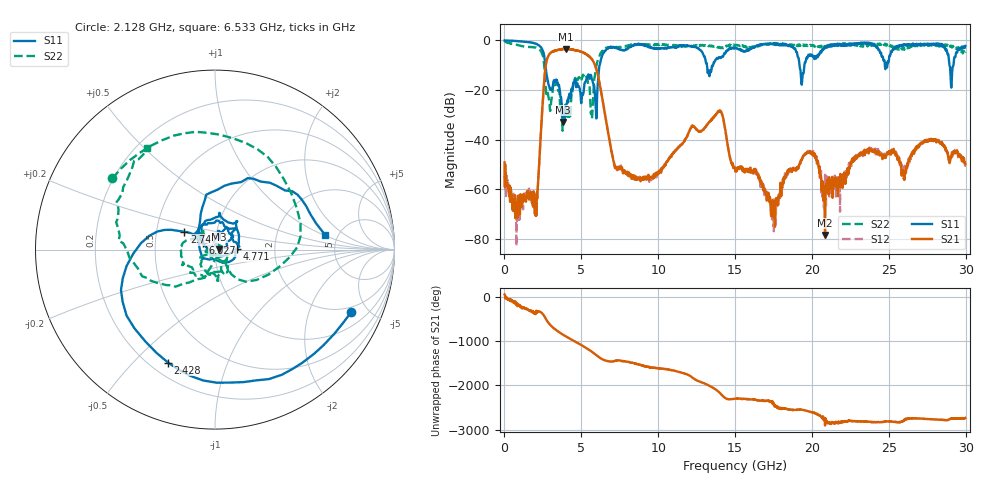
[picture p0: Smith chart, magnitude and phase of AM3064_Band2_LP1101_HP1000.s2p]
# Hz S DB R 50.0
!freq dBS11 angS11 dBS21 angS21 dBS12 angS12 dBS22 angS22
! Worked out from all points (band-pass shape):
!   1600 points, 10 MHz to 29.98 GHz, reference 50 ohm
!   highest |S21| = -3.45 dB at 4.002 GHz (marker M1); lowest = -78.4 dB at 20.85 GHz (marker M2)
!   |S21| within 3 dB of the highest: 2.842 GHz to 5.521 GHz (2.679 GHz wide, 64.1 % of centre)
!   lowest |S11| = -32.9 dB at 3.815 GHz (marker M3), VSWR 1.05, Z = 52.3 + j0.384 ohm
!   |S11| at or under -10 dB: 2.663 GHz to 6.193 GHz (3.53 GHz wide, 79.7 % of centre); 13.17 GHz to 13.57 GHz (398 MHz wide, 2.98 % of centre); 19.19 GHz to 19.51 GHz (324.4 MHz wide, 1.68 % of centre)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
!   |S22| runs from -36.4 to -0.3 dB; largest |S21 - S12| = 0.015
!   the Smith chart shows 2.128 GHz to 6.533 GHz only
!   S11 on the Smith chart (normalised r, x): 2.128 GHz: 1.68, -3.86; 2.428 GHz: 0.27, -0.63; 2.747 GHz: 0.70, +0.14; 4.771 GHz: 1.27, +0.01; 6.027 GHz: 0.87, +0.06; 6.533 GHz: 3.95, +1.05
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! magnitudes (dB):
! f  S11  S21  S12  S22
! 10 MHz  -0.1  -49.2  -54.5  -0.3
! 816 MHz  -0.3  -68.1  -72.8  -1.8
! 2.128 GHz  -1.6  -63.8  -60.8  -3.2
! 2.428 GHz  -3.3  -31.1  -31.1  -5.2
! 2.747 GHz  -14.1  -8.1  -8.1  -21.1
! 3.815 GHz  -32.9  -3.5  -3.5  -30.6
! 4.002 GHz  -26.0  -3.4  -3.5  -28.9
! 4.771 GHz  -18.4  -4.3  -4.1  -15.9
! 5.015 GHz  -24.0  -4.6  -4.7  -15.8
! 5.671 GHz  -15.4  -7.5  -7.5  -30.2
! 6.027 GHz  -22.3  -12.7  -12.6  -9.0
! 6.533 GHz  -4.2  -29.5  -29.4  -3.4
! 7.283 GHz  -3.2  -51.7  -52.0  -2.6
! 10 GHz  -3.3  -53.7  -53.3  -1.8
! 13.97 GHz  -6.8  -28.8  -28.4  -2.9
! 15 GHz  -2.9  -52.1  -51.3  -1.9
! 17.5 GHz  -1.6  -69.2  -70.6  -1.2
! 19.99 GHz  -5.7  -45.4  -45.4  -1.9
! 20.85 GHz  -3.1  -78.4  -54.2  -2.4
! 25 GHz  -8.3  -44.8  -45.4  -1.6
! 29.08 GHz  -17.8  -46.2  -46.7  -2.5
! 29.98 GHz  -2.3  -49.9  -50.1  -4.7
